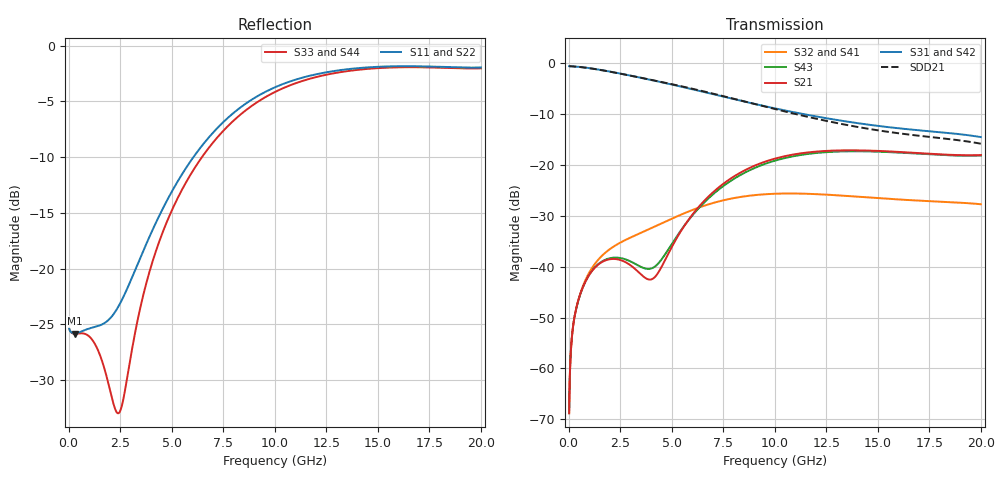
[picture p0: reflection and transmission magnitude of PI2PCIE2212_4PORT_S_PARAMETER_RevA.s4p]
! NPort=4 DATA=800 NOISE=0 GROUPDELAY=0 COMPLEX_DATAFORMAT=POLAR
! NumOfBlock=1 NumOfParam=0
! .MODEL Smodel S TSTONEFILE=PI2PCIE2212_4PORT_S_PARAMETER_RevA.s4p TYPE=S
!  -- The above .MODEL line can be used for the S element in the netlist.
! PORT DEFINITION
! PORT1 = INPUT+
! PORT2 = INPUT-
! PORT3 = OUTPUT+
! PORT4 = OUTPUT-
# Hz S MA R  50
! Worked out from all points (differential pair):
!   800 points, 25 MHz to 20 GHz, reference 50 ohm
!   strongest paths, dB at 25 MHz, 5.025 GHz, 10.03 GHz, 15.03 GHz, 20 GHz:
!     S31: -0.5, -4.2, -8.9, -12.3, -14.5
!     S42: -0.5, -4.2, -8.9, -12.3, -14.5
!     S21: -68.8, -36.0, -18.7, -17.2, -18.0
!     S43: -68.8, -35.4, -19.1, -17.4, -18.1
!     S32: -68.8, -30.5, -25.6, -26.5, -27.7
!     S41: -68.8, -30.5, -25.6, -26.5, -27.7
!   taken as a pair (ports 1,2 in; 3,4 out), SDD21 dB: -0.5, -4.1, -9.0, -13.2, -15.8
!   lowest |S11| = -25.8 dB at 300 MHz (marker M1), VSWR 1.11, Z = 55.2 - j1.53 ohm
!   |S11| at or under -10 dB: start of sweep to 6.052 GHz
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2.5e7  0.05397 -3.1  0.000363 86.7  0.9398 -0.7  0.0003616 86.7
       0.000363 86.7  0.05396 -3.1  0.0003616 86.7  0.9398 -0.7
       0.9398 -0.7  0.0003616 86.7  0.05403 -2.4  0.000363 86.8
       0.0003616 86.7  0.9398 -0.7  0.000363 86.8  0.05404 -2.4
3e8  0.05123 -15.7  0.00332 69.4  0.9323 -6.7  0.003323 69.0
     0.00332 69.4  0.05121 -15.8  0.003323 69.0  0.9323 -6.7
     0.9323 -6.7  0.003323 69.0  0.05105 -8.1  0.003318 69.7
     0.003323 69.0  0.9323 -6.7  0.003318 69.7  0.05107 -8.1
2.45e9  0.06859 -159.6  0.01173 44.3  0.799 -48.0  0.01702 37.3
        0.01174 44.3  0.06895 -159.6  0.01702 37.3  0.7989 -48.0
        0.799 -48.0  0.01702 37.3  0.0226 -150.8  0.01224 48.2
        0.01702 37.3  0.7988 -48.0  0.01224 48.2  0.02259 -151.0
4.125e9  0.153 112.0  0.007721 88.8  0.6792 -74.9  0.02457 20.1
         0.007721 88.7  0.1534 112.1  0.02457 20.2  0.679 -74.9
         0.6792 -74.8  0.02457 20.2  0.1117 91.3  0.009851 84.2
         0.02457 20.1  0.6789 -74.9  0.009849 84.2  0.1118 91.2
7.8e9  0.4817 14.0  0.07228 104.7  0.4559 -124.4  0.04642 -31.7
       0.07227 104.7  0.4819 14.0  0.04642 -31.7  0.4558 -124.3
       0.456 -124.4  0.04642 -31.7  0.443 8.7  0.06853 101.1
       0.04642 -31.7  0.4557 -124.4  0.06854 101.1  0.4433 8.7
1.3375e10  0.7817 -62.5  0.1397 36.9  0.2703 177.9  0.04991 -120.2
           0.1397 36.9  0.7817 -62.5  0.04991 -120.2  0.2704 178.0
           0.2704 178.0  0.04991 -120.2  0.7661 -63.2  0.1364 37.1
           0.04991 -120.2  0.2703 178.0  0.1364 37.1  0.7664 -63.2
2e10  0.799 -97.7  0.1255 5.7  0.1883 100.6  0.04118 146.2
      0.1255 5.7  0.7992 -97.7  0.04118 146.2  0.1884 100.7
      0.1884 100.6  0.04118 146.2  0.7922 -97.9  0.1241 6.1
      0.04118 146.2  0.1883 100.6  0.1241 6.1  0.7922 -97.9
